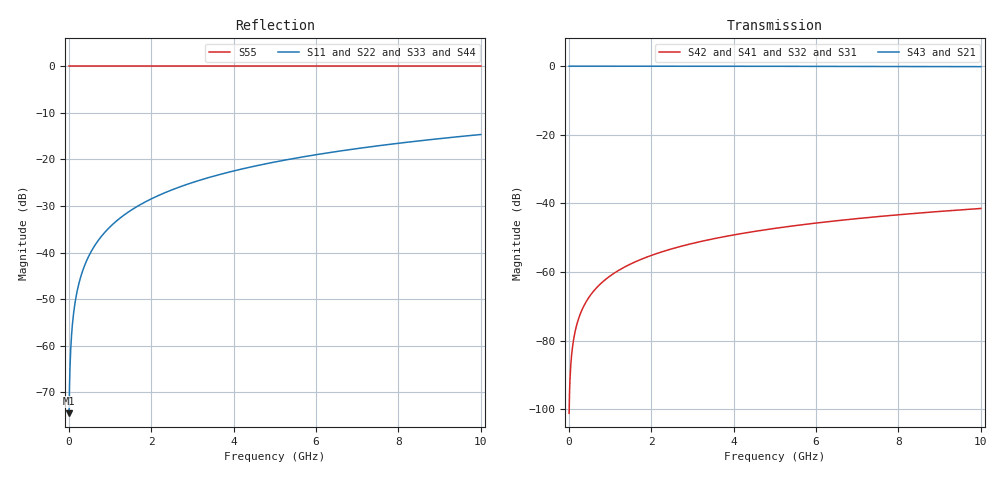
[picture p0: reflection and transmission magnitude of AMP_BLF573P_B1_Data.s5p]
! Created Mon Jul 19 16:24:23 2010
# ghz S ma R 50
! 5 Port Network Data from SP1.SP block
! freq  magS11  angS11  magS12  angS12  magS13  angS13  magS14  angS14
!  magS15  angS15
!  magS21  angS21  magS22  angS22  magS23  angS23
!  magS24  angS24  magS25  angS25
!  magS31  angS31  magS32  angS32
!  magS33  angS33  magS34  angS34  magS35  angS35
!  magS41  angS41
!  magS42  angS42  magS43  angS43  magS44  angS44  magS45  angS45
!  magS51  angS51  magS52  angS52  magS53  angS53  magS54  angS54
!  magS55  angS55
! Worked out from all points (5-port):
!   1000 points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, 10 MHz to 10 GHz, reference 50 ohm
!   strongest paths, dB at 10 MHz, 2.51 GHz, 5.01 GHz, 7.51 GHz, 10 GHz:
!     S43: 0.0, 0.0, 0.0, -0.1, -0.1
!     S21: 0.0, 0.0, 0.0, -0.1, -0.2
!     S42: -101.2, -53.2, -47.3, -43.8, -41.5
!     S41: -101.2, -53.2, -47.3, -43.8, -41.5
!     S32: -101.2, -53.2, -47.3, -43.8, -41.5
!     S31: -101.2, -53.2, -47.3, -43.8, -41.5
!   lowest |S11| = -74.5 dB at 10 MHz (marker M1), VSWR 1.00, Z = 50 + j0.0188 ohm
!   |S11| at or under -10 dB: start of sweep to end of sweep
